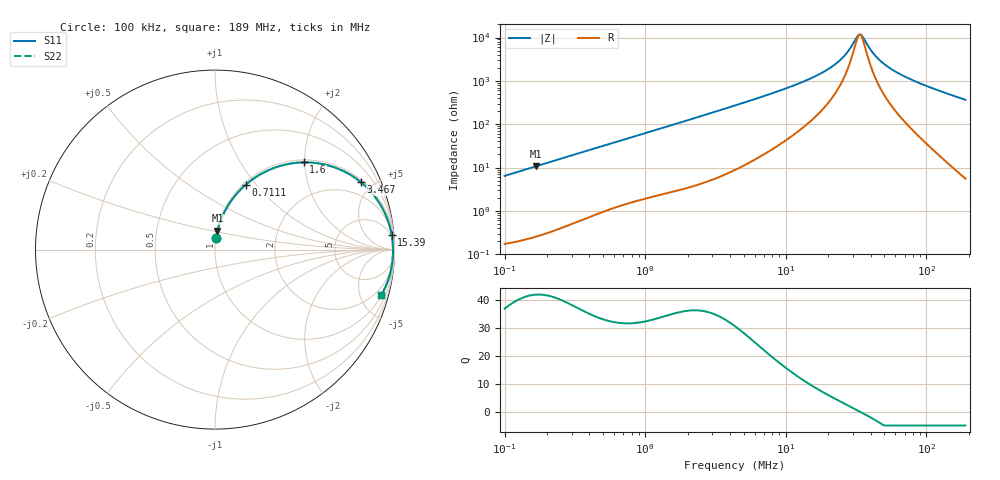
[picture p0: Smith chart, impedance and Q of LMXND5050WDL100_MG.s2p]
! LMXND5050WDL100_MG  S-PARAMETER MODEL  ( General Type )
! Model Generated by TAIYO YUDEN Corporation (http://www.ty-top.com)
! Version 1.0
! TAIYO YUDEN Control No. 191023NI43SB-FBB
! Copyright(c) 2019 TAIYO YUDEN CO.,LTD. All Rights Reserved.
! Product Description (link to TY-COMPAS)
! https://ds.yuden.co.jp/TYCOMPAS/or/detail?pn=LMXND5050WDL100MMG&u=M
! Products Name : Inductors
! Characteristics :
!  Inductance : 10 uH , SRF(min) : 21 MHz , DC Resistance(max) : 0.15 Ohm
!  Rated Current : Saturation :1700 mA , Temp Rise : 1200 mA
!  Case Size : 4.9 x 4.9 / 0.193 x 0.193 [mm/inch] , Thickness : 2.4 / 0.094 [mm/inch]
!  (Conditions: Temperature = 25 degC , DC Bias Current/Voltage = 0A / 0V)
! External Node Assignments :
!  1  o---GGG---o  2
! GND o---------o GND
! Frequency Range : 0.1MHz  -  189.042664MHz  [ 402 STEP ]
# MHz S RI R 50
! Freq[MHz].  S11 Real  S11 Imag  S21 Real  S21 Imag  S12 Real  S12 Imag  S22 Real  S22 Imag
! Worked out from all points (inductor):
!   401 points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, 100 kHz to 189 MHz, reference 50 ohm
!   read as one part in series: L = 10.2 uH near 103.8 kHz
!   highest Q = 42.1 at 166.4 kHz (marker M1), where L = 10.2 uH
!   self-resonance near 33.34 MHz
!   S11 on the Smith chart (normalised r, x): 100 kHz: 1.00, +0.13; 711.1 kHz: 1.03, +0.89; 1.6 MHz: 1.06, +1.97; 3.467 MHz: 1.13, +4.28; 15.39 MHz: 4, +23; 189 MHz: 1.11, -7.31
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0.1  0.00578 0.0635  0.9942 -0.0635  0.9942 -0.0635  0.00578 0.0635
0.166406  0.0136 0.1046  0.9864 -0.1046  0.9864 -0.1046  0.0136 0.1046
0.353854  0.0532 0.2112  0.9468 -0.2112  0.9468 -0.2112  0.0532 0.2112
0.711059  0.1727 0.3626  0.8273 -0.3626  0.8273 -0.3626  0.1727 0.3626
1.252125  0.3781 0.4703  0.6219 -0.4703  0.6219 -0.4703  0.3781 0.4703
1.600058  0.4932 0.486  0.5068 -0.486  0.5068 -0.486  0.4932 0.486
2.246885  0.6526 0.4626  0.3474 -0.4626  0.3474 -0.4626  0.6526 0.4626
3.467234  0.8139 0.3748  0.1861 -0.3748  0.1861 -0.3748  0.8139 0.3748
4.347904  0.8715 0.3188  0.1285 -0.3188  0.1285 -0.3188  0.8715 0.3188
9.072866  0.9639 0.1599  0.0361 -0.1599  0.0361 -0.1599  0.9639 0.1599
15.38522  0.9841 0.0821  0.0159 -0.0821  0.0159 -0.0821  0.9841 0.0821
20.03472  0.9885 0.0517  0.0115 -0.0517  0.0115 -0.0517  0.9885 0.0517
24.19342  0.9903 0.032  0.00973 -0.032  0.00973 -0.032  0.9903 0.032
27.09229  0.991 0.0208  0.00904 -0.0208  0.00904 -0.0208  0.991 0.0208
32.10467  0.9915 0.00431  0.00847 -0.00431  0.00847 -0.00431  0.9915 0.00431
33.33888  0.9916 0.000678  0.00841 -0.000678  0.00841 -0.000678  0.9916 0.000678
35.27973  0.9916 -0.00477  0.00837 0.00477  0.00837 0.00477  0.9916 -0.00477
40.25919  0.9915 -0.0176  0.0085 0.0176  0.0085 0.0176  0.9915 -0.0176
44.24071  0.9912 -0.027  0.00878 0.027  0.00878 0.027  0.9912 -0.027
54.44117  0.9899 -0.0485  0.0101 0.0485  0.0101 0.0485  0.9899 -0.0485
88.90043  0.9813 -0.1096  0.0187 0.1096  0.0187 0.1096  0.9813 -0.1096
189.0427  0.9271 -0.2525  0.0729 0.2525  0.0729 0.2525  0.9271 -0.2525
